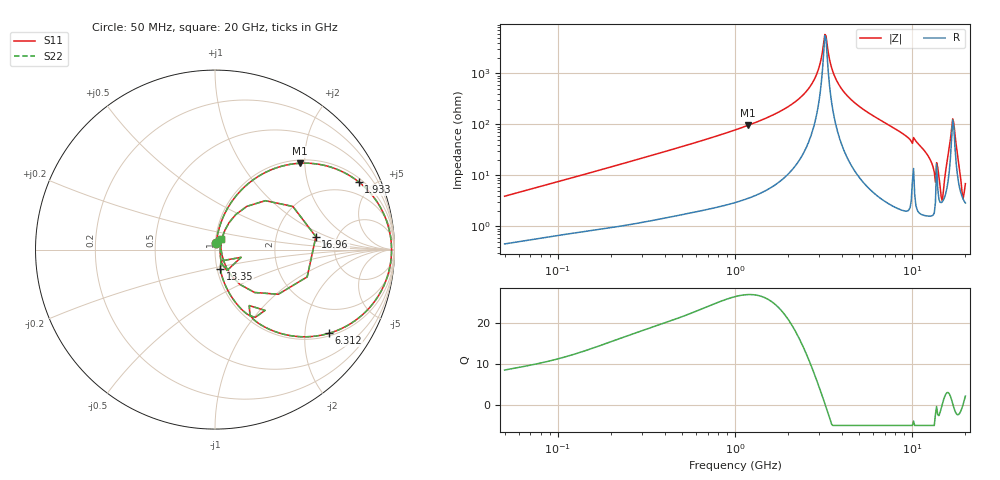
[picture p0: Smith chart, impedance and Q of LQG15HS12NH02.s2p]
!Murata Part Number: LQG15HS12NH02
!These Parameters are Measured in Series Mode Connection
!  o--[Z]--o
!Port1  Port2
!  o-------o
!Freq. Start=50[MHz] Stop=20[GHz], 401[Steps]
# Hz S RI R 50
!Freq.(Hz) S11(Real) S11(Imag) S21(Real) S21(Imag) S12(Real) S12(Imag) S22(Real) S22(Imag)
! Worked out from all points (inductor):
!   401 points, 50 MHz to 20 GHz, reference 50 ohm
!   read as one part in series: L = 12.2 nH near 51.52 MHz
!   highest Q = 27 at 1.179 GHz (marker M1), where L = 12.8 nH
!   self-resonance near 3.217 GHz
!   S11 on the Smith chart (normalised r, x): 50 MHz: 1.01, +0.08; 1.933 GHz: 1.19, +4.13; 6.312 GHz: 1.08, -2.66; 13.35 GHz: 1.04, -0.23; 16.96 GHz: 3.45, +0.73; 20 GHz: 1.06, +0.12
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5e7  0.00599 0.0383  0.994 -0.0383  0.994 -0.0383  0.00599 0.0383
1.364002e8  0.0176 0.0983  0.9824 -0.0983  0.9824 -0.0983  0.0176 0.0983
3.721004e8  0.079 0.2455  0.921 -0.2455  0.921 -0.2455  0.079 0.2455
1e9  0.379 0.4666  0.621 -0.4666  0.621 -0.4666  0.379 0.4666
1.179116e9  0.4744 0.4811  0.5256 -0.4811  0.5256 -0.4811  0.4744 0.4811
1.932977e9  0.7998 0.3778  0.2002 -0.3778  0.2002 -0.3778  0.7998 0.3778
2.728004e9  0.9602 0.1474  0.0398 -0.1474  0.0398 -0.1474  0.9602 0.1474
2.98453e9  0.9783 0.0713  0.0217 -0.0713  0.0217 -0.0713  0.9783 0.0713
3.168813e9  0.9834 0.0186  0.0166 -0.0186  0.0166 -0.0186  0.9834 0.0186
3.265178e9  0.9837 -0.0081  0.0163 0.0081  0.0163 0.0081  0.9837 -0.0081
3.572216e9  0.9759 -0.0885  0.0241 0.0885  0.0241 0.0885  0.9759 -0.0885
3.967106e9  0.9495 -0.1804  0.0505 0.1804  0.0505 0.1804  0.9495 -0.1804
6.311513e9  0.6358 -0.4663  0.3642 0.4663  0.3642 0.4663  0.6358 -0.4663
7.442007e9  0.4765 -0.4854  0.5235 0.4854  0.5235 0.4854  0.4765 -0.4854
1.066139e10  0.1739 -0.3555  0.8261 0.3555  0.8261 0.3555  0.1739 -0.3555
1.334722e10  0.0301 -0.108  0.9699 0.108  0.9699 0.108  0.0301 -0.108
1.482269e10  0.0296 0.00667  0.9704 -0.00667  0.9704 -0.00667  0.0296 0.00667
1.621653e10  0.177 0.2409  0.823 -0.2409  0.823 -0.2409  0.177 0.2409
1.696185e10  0.5621 0.072  0.4379 -0.072  0.4379 -0.072  0.5621 0.072
1.774144e10  0.2208 -0.239  0.7792 0.239  0.7792 0.239  0.2208 -0.239
1.912117e10  0.0384 -0.0279  0.9616 0.0279  0.9616 0.0279  0.0384 -0.0279
2e10  0.0315 0.0588  0.9685 -0.0588  0.9685 -0.0588  0.0315 0.0588
